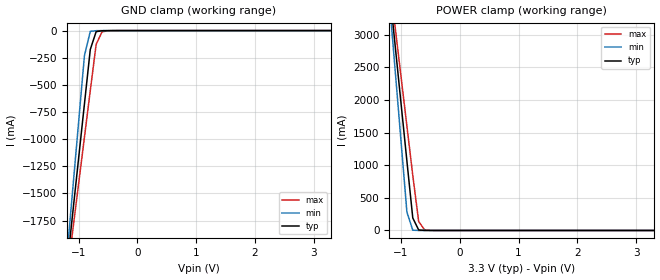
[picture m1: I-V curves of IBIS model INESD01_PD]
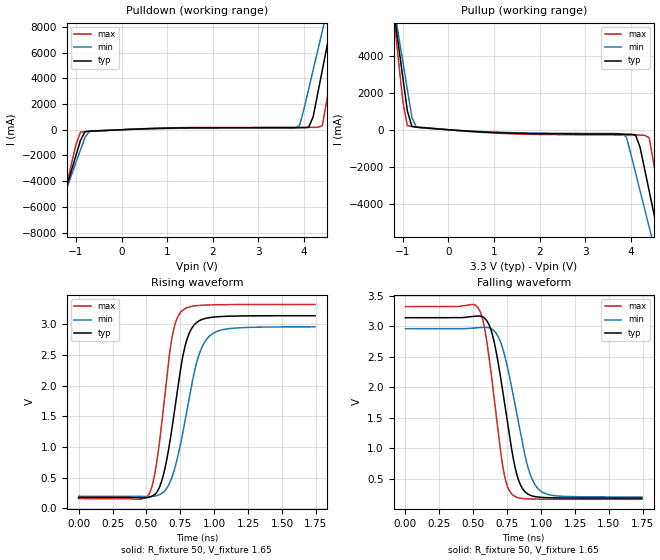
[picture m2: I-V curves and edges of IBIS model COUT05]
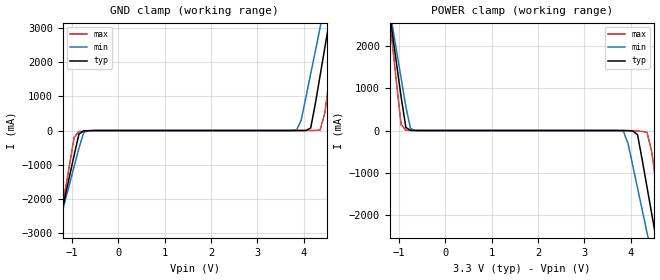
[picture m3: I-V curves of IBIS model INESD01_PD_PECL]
|   This file is an IBIS representation of the   |
|   Integrated Device Technology , Inc.   |
|   ICS87950I   |
|   LOW SKEW, 1-TO-9 LVCMOS/LVTTL Clock Multiplier   |
[IBIS Ver]   4.1
[File name]   87950i_3v3.ibs
[File Rev]   1.0
[Date]   22 Jun 2009 | Last modified
[Source]   Originated at Integrated Device Technology, Inc.
[Disclaimer]
IDT hereby grants the user of this IBIS model a non-exclusive,
nontransferable license to use this IBIS model under the following terms.
Before using this IBIS model, the user should read this license.
If the user does not accept these terms,  the IBIS model should be
returned to IDT within 30 days.
   The user is granted this license only to use the IBIS model and
is not granted rights to sell, load, rent, lease or license the IBIS
model in whole or in part, or in modified form to anyone other than
user. User may modify the IBIS model to suit its specific
applications but rights to derivative works and such modifications
shall belong to IDT.
   This IBIS model is provided on an "AS IS" basis and IDT makes
absolutely no warranty with respect to the information contained
herein. IDT DISCLAIMS AND CUSTOMER WAIVES ALL WARRANTIES, EXPRESS
OR IMPLIED, INCLUDING WARRANTIES OF MERCHANTABILITY OR FITNESS FOR
A PARTICULAR PURPOSE. The entire risk as to quality and performance
is with the Customer. ACCORDINGLY, IN NO EVENT SHALL THE COMPANY BE
LIABLE FOR ANY DAMAGES, WHETHER IN CONTRACT OR TORT,INCLUDING ANY
LOST PROFITS OR OTHER INCIDENTAL, CONSEQUENTIAL, EXEMPLARY, OR
PUNITIVE DAMAGES ARISING OUT OF THE USE OR APPLICATION OF THE IBIS
model provided in this package. Further, IDT reserves the right to
make changes without notice to any product herein to improve
reliability, function, or design. IDT does not convey any license
under patent rights or any other intellectual property rights,
including those of third parties.
   IDT is not obligated to provide maintenance or support
for the licensed IBIS model.
[Copyright]   Copyright 2003 by Integrated Device Technology , Inc.
[Component]   ICS87950i
[Manufacturer] Integrated Device Technology, Inc.
[Package]
|LQFP32
|lead + wire   typ   min   max
R_pkg   220.4m   212.5m   238m
L_pkg   1.841nH   1.708nH   1.974n
C_pkg   0.316pF   0.2907pF   0.33pF
[Pin] signal_name   model_name   R_pin   L_pin   C_pin
1   VDDA   POWER   238m   1.974n   0.330p
2   FBDIV_SEL   INESD01_PD   225m   1.841n   0.311p
3   DIV_SELA   INESD01_PD   218m   1.7745n   0.301p
4   DIV_SELB   INESD01_PD   213m   1.708n   0.291p
5   DIV_SELC   INESD01_PD   213m   1.708n   0.291p
6   DIV_SELD   INESD01_PD   218m   1.7745n   0.301p
7   GND   GND   225m   1.841n   0.311p
8   XTAL_IN   NC   238m   1.974n   0.330p
9   XTAL_OUT   NC   238m   1.974n   0.330p
10   MR/nOE   INESD01_PD   225m   1.841n   0.311p
11   VDDO   POWER   218m   1.7745n   0.301p
12   QD4   COUT05   213m   1.708n   0.291p
13   GND   GND   213m   1.708n   0.291p
14   QD3   COUT05   218m   1.7745n   0.301p
15   VDDO   POWER   225m   1.841n   0.311p
16   QD2   COUT05   238m   1.974n   0.330p
17   GND   GND   238m   1.974n   0.330p
18   QD1   COUT05   225m   1.841n   0.311p
19   VDDO   POWER   218m   1.7745n   0.301p
20   QD0   COUT05   213m   1.708n   0.291p
21   GND   GND   213m   1.708n   0.291p
22   QC1   COUT05   218m   1.7745n   0.301p
23   VDDO   POWER   225m   1.841n   0.311p
24   QC0   COUT05   238m   1.974n   0.330p
25   GND   GND   238m   1.974n   0.330p
26   QB   COUT05   225m   1.841n   0.311p
27   VDDO   POWER   218m   1.7745n   0.301p
28   QA   COUT05   213m   1.708n   0.291p
29   GND   GND   213m   1.708n   0.291p
30   CLK   INESD01_PD_PECL   218m   1.7745n   0.301p
31   PLL_SEL   INESD01_PD   225m   1.841n   0.311p
32   CLK_SEL   INESD01_PD   238m   1.974n   0.330p
| Models and submodels in the file (3): INESD01_PD (Input), COUT05 (Output), INESD01_PD_PECL (Input)
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[Model]   INESD01_PD
Model_type   Input
Polarity   Non-Inverting
Vinl = 0.80V
Vinh = 2.0V
|   typ   min   max
C_comp   2pF   1.5pF   2.5pF
|   typ   min   max
[Voltage range]  3.3V   3.15V   3.45V
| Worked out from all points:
|   GND clamp passes 1 mA (typ) near -0.55 V on its own axis
|   POWER clamp passes 1 mA (typ) near -0.60 V on its own axis
[GND_clamp]
|Voltage I(typ)   I(min)   I(max)
-3.3V     -12.83A    -15.14A    -11.37A
-1.2V     -2.195A    -2.092A    -2.281A
-1.1V     -1.689A    -1.472A    -1.849A
-900mV    -678.5mA   -232.6mA   -984.8mA
-800mV    -173.9mA   -7.175mA   -553.2mA
-700mV    -9.696mA   -1.052mA   -126mA
-600mV    -1.629mA   -178uA     -11.07mA
-300mV    -10.53uA   -5.678uA   -86.08uA
3.3V      71.13uA    62.11uA    77.58uA
[POWER_clamp]
|Voltage   I(typ)   I(min)   I(max)
-3.3V     22.38A     26.45A     19.82A
-1.2V     3.723A     3.545A     3.874A
-1.1V     2.836A     2.457A     3.116A
-1V       1.949A     1.369A     2.358A
-900mV    1.063A     281.1mA    1.601A
-800mV    191.6mA    5.074mA    844mA
-700mV    8.104mA    204.3uA    138.4mA
-600mV    678.1uA    79.74uA    10.7mA
-400mV    87.44uA    69.65uA    413.2uA
3.3V      -3.041nA   -425fA     -919.9nA
[Model]   COUT05
Model_type   Output
Polarity   Non-Inverting
|   typ   min   max
C_comp   2pF   1.5pF   2.5pF
Vmeas = 1.65V
Rref = 50
Cref = 0
Vref = 1.65V
|   typ   min   max
[Voltage range]   3.3V   3.135V   3.465V
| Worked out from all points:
|   slope of the pulldown table from 0 to 0.495 V, typ, clamps not added: 6.88 ohm
|   slope of the pullup table from 0 to 0.495 V, typ, clamps not added: 5.83 ohm
|   rising waveform, R_fixture 50, V_fixture 1.65: 20-80 % time 127ps typ, 154ps min, 103ps max; typ from 0.181 V to 3.14 V
|   falling waveform, R_fixture 50, V_fixture 1.65: 20-80 % time 128ps typ, 151ps min, 107ps max; typ from 3.14 V to 0.181 V
[Pulldown]
|Voltage   I (typ)   I (min)   I (max)
-3.3V     -29.26A    -25.28A    -35.95A
-1.5V     -7.949A    -7.508A    -8.752A
-900mV    -829.9mA   -1.575A    -187.1mA
-700mV    -111.2mA   -118.1mA   -127.5mA
3.9V      159.4mA    311mA      182.9mA
4.1V      184.8mA    3.152A     184mA
4.2V      1.015A     4.66A      185mA
4.4V      4.637A     7.679A     308.5mA
4.6V      8.262A     10.7A      4.646A
4.7V      10.08A     12.21A     6.964A
4.8V      11.89A     13.72A     9.282A
6.6V      44.81A     41.14A     51.33A
[Pullup]
|Voltage   I (typ)   I (min)   I (max)
-3.3V     44.73A     38.61A     55.03A
-1.2V     6.49A      6.732A     6.202A
-1.1V     4.667A     5.214A     3.875A
-900mV    1.021A     2.176A     220.8mA
-700mV    135.9mA    139mA      157.7mA
3.8V      -238.9mA   -217.3mA   -279.5mA
4.1V      -276.1mA   -2.314A    -283.5mA
4.3V      -2.128A    -4.28A     -299.6mA
4.4V      -3.308A    -5.264A    -428.8mA
4.6V      -5.67A     -7.233A    -3.347A
4.8V      -8.032A    -9.203A    -6.363A
6.6V      -29.3A     -26.93A    -33.51A
[Ramp]
|   typ   min   max
dV/dt_r   2.374/0.197n   2.212/0.24n   2.539/0.159n
dV/dt_f   2.39/0.193n   2.226/0.229n   2.557/0.16n
R_load =   50.0000
[Rising Waveform]
R_fixture = 50
V_fixture = 1.65   |Vcc_typ
V_fixture_min = 1.5675 |Vcc_min
V_fixture_max = 1.7325 |Vcc_max
C_fixture = 0.0p
| Time   typ   min   max
0s        180.7mV    199.5mV    160.8mV
520.5ps   183.7mV    193.6mV    238.7mV
572.6ps   253.4mV    207.2mV    702.8mV
631.1ps   597.9mV    276.8mV    1.746V
696.2ps   1.42V      560mV      2.869V
767.8ps   2.469V     1.228V     3.231V
813.3ps   2.843V     1.767V     3.282V
878.4ps   3.043V     2.438V     3.306V
976ps     3.113V     2.83V      3.317V
1.744ns   3.14V      2.96V      3.323V
[Falling Waveform]
R_fixture = 50
V_fixture = 1.65   |Vcc_typ
V_fixture_min = 1.5675 |Vcc_min
V_fixture_max = 1.7325 |Vcc_max
C_fixture = 0.0p
| Time   typ   min   max
0s        3.141V     2.96V      3.323V
540ps     3.169V     2.979V     3.285V
585.6ps   3.128V     2.983V     2.941V
644.1ps   2.836V     2.942V     2.006V
722.2ps   1.868V     2.597V     639.8mV
793.8ps   843.8mV    1.879V     227.6mV
839.3ps   443.3mV    1.347V     182.7mV
904.4ps   245.1mV    677.6mV    167.6mV
995.5ps   194mV      299.1mV    162.9mV
1.744ns   180.7mV    199.6mV    160.8mV
[Model]   INESD01_PD_PECL
Model_type  Input
Polarity   Non-Inverting
Vinl = 0.8V
Vinh = 2.0V
|   typ   min   max
C_comp   2pF   1.5pF   2.5pF
|   typ   min   max
[Voltage range]  3.3V   3.15V   3.45V
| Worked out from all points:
|   GND clamp passes 1 mA (typ) near -0.55 V on its own axis
|   POWER clamp passes 1 mA (typ) near -0.66 V on its own axis
[GND_clamp]
|Voltage   I(typ)   I(min)   I(max)
-2.586V   -10.86A    -9.487A    -13.15A
-1.361V   -3.24A     -3.145A    -3.432A
-1.259V   -2.606A    -2.617A    -2.622A
-952.6mV  -705.3mA   -1.038A    -192.4mA
-850.5mV  -99.9mA    -513.5mA   -31.23mA
-646.4mV  -3.788mA   -3.549mA   -8.297mA
3.844V    129.1uA    13.13mA    71.12uA
4.151V    73.33mA    1.652A     864.7uA
4.355V    1.607A     3.003A     15.44mA
4.559V    3.233A     4.356A     1.553A
4.763V    4.861A     5.711A     3.635A
5.375V    9.757A     9.783A     9.893A
[POWER_clamp]
|Voltage   I(typ)   I(min)   I(max)
-2.177V   10.57A     9.364A     12.62A
-1.157V   2.42A      2.586A     2.194A
-952.6mV  795.8mA    1.237A     137.8mA
-850.5mV  73.33mA    563.2mA    8.145mA
-646.4mV  535.8uA    2.004mA    431.2uA
3.844V    -826.3uA   -18.14mA   -47.07uA
4.151V    -99.9mA    -1.362A    -11.82mA
4.355V    -1.338A    -2.415A    -41.71mA
4.559V    -2.606A    -3.47A     -1.312A
4.661V    -3.24A     -3.998A    -2.123A
4.763V    -3.875A    -4.526A    -2.933A
5.579V    -8.954A    -8.756A    -9.414A
